PROGRAM MAIN
VAR CONSTANT	
	cInitSource		: ST_MA_MultiArray_InitPars 	
						:= ( eTypeCode := eMA_TypeCode_LREAL, nDims := 2, aDimSizes := [cChannels, cBufferLength]);													 				 
END_VAR

VAR	
	nInputSelection		: UDINT := 1;
	aCrestFactor		: ARRAY[1..cChannels] OF LREAL;		
	nSampleIdx			: UDINT;
	nChannelIdx			: UDINT;				
	aEl3632 AT %I*		: ARRAY[1..cChannels] OF ARRAY[1..cOversamples] OF INT;		// input from hardware e.g. EL3632
	aBuffer				: ARRAY[1..cChannels] OF ARRAY[1..cOversamples] OF LREAL;		
	
	fbSource			: FB_CMA_Source := (stInitPars := cInitSource, nOwnID := eID_Source, aDestIDs := [eID_Crest]);	// Initialize source					
	fbSink				: FB_CMA_Sink := (nOwnID := eID_Sink);		
	
	aFunctionGenerator	: ARRAY[1..cChannels] OF FB_FunctionGenerator;	
	fSetFrequency		: LREAL := 20; 		// Hz
	fSetAmplitude		: LREAL := 5;		// peak amplitude of sin signal		
	fbErrHist			: FB_HRErrHist; 	// error monitoring
	bNewResult			: BOOL;
END_VAR

FOR nChannelIdx := 1 TO cChannels DO
	CASE nInputSelection OF
		0:  (* input from EL3632 *)
			FOR nSampleIdx := 1 TO cOversamples DO
				aBuffer[nChannelIdx][nSampleIdx] := INT_TO_LREAL(aEl3632[nChannelIdx][nSampleIdx]);
			END_FOR
	
		1:  (* signal generator *)		
			aFunctionGenerator[nChannelIdx](	bEnable		:= TRUE,
												fFrequency 	:= fSetFrequency,
												fAmplitude 	:= fSetAmplitude,												
												eFunction 	:= E_FunctionType.Sine,
												aSignal		:= aBuffer[nChannelIdx] );
	END_CASE
END_FOR						

// Collect data in a source	
fbSource.Input2DStd(	pDataIn 			:= ADR(aBuffer),
						nDataInSize 		:= SIZEOF(aBuffer), 
						eElementType 		:= eMA_TypeCode_LREAL,
						nOptionPars			:= 0 );	  
IF fbSource.bError THEN
	fbErrHist.AddError(bErr:=TRUE, hrErrCode:=fbSource.hrErrorCode, sErrSource:='MAIN.fbSource'); // error monitoring
	//ToDo: if error
END_IF

// Push results to sink
fbSink.Output1DStd( 	pDataOut 		:= ADR(aCrestFactor), 
						nDataOutSize 	:= SIZEOF(aCrestFactor), 
						eElementType 	:= eMA_TypeCode_LREAL, 
						nOptionPars		:= 0,
						bNewResult		=> bNewResult);	
IF fbSink.bError THEN
	fbErrHist.AddError(bErr:=TRUE, hrErrCode:=fbSink.hrErrorCode, sErrSource:='MAIN.fbSink'); // error monitoring
	//ToDo: if error
END_IF
IF bNewResult THEN
	// ToDo: if the buffer is ready
END_IF

END_PROGRAM
